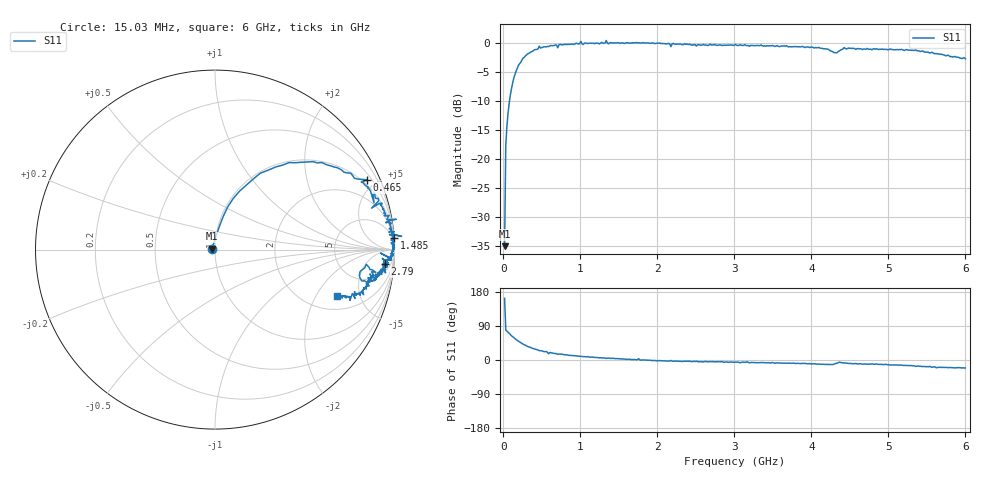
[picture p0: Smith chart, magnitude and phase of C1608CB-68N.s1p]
!	Network	Analyzer	HP8753E.07.74:	Oct	30	2002	Serial	No.	JP38451487
!	Hewlett-Packard
!	7	Sep	2009	9:48:31
!	Frequency	S11
#	HZ	S	RI	R	50
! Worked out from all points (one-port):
!   400 points, 15.03 MHz to 6 GHz, reference 50 ohm
!   lowest |S11| = -35.0 dB at 15.03 MHz (marker M1), VSWR 1.04, Z = 48.3 + j0.512 ohm
!   |S11| at or under -10 dB: start of sweep to 79.43 MHz
!   S11 on the Smith chart (normalised r, x): 15.03 MHz: 0.97, +0.01; 465 MHz: 0.74, +4.46; 1.485 GHz: -0, +30; 2.79 GHz: 10, -17; 6 GHz: 2.77, -3.02
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1.502992e7  -0.0169 0.00529
3.002985e7  0.0235 0.127
6.00297e7  0.0709 0.238
9.002955e7  0.138 0.327
1.95029e8  0.414 0.485
4.650277e8  0.848 0.389
5.550272e8  0.85 0.349
5.850271e8  0.886 0.261
6.150269e8  0.889 0.315
7.650262e8  0.921 0.251
1.005025e9  1.01 0.169
1.035025e9  0.951 0.15
1.335023e9  1.04 0.0732
1.365023e9  0.972 0.0837
1.485023e9  0.998 0.0661
1.515022e9  0.981 0.0529
1.755021e9  0.993 0.0632
2.145019e9  0.982 -0.0492
2.175019e9  0.922 -0.0194
2.265019e9  0.973 -0.0511
2.790016e9  0.947 -0.0813
3.015015e9  0.959 -0.0962
3.765011e9  0.911 -0.131
4.305008e9  0.804 -0.146
4.365008e9  0.843 -0.0819
4.515007e9  0.883 -0.142
5.265004e9  0.833 -0.219
6e9  0.677 -0.259
